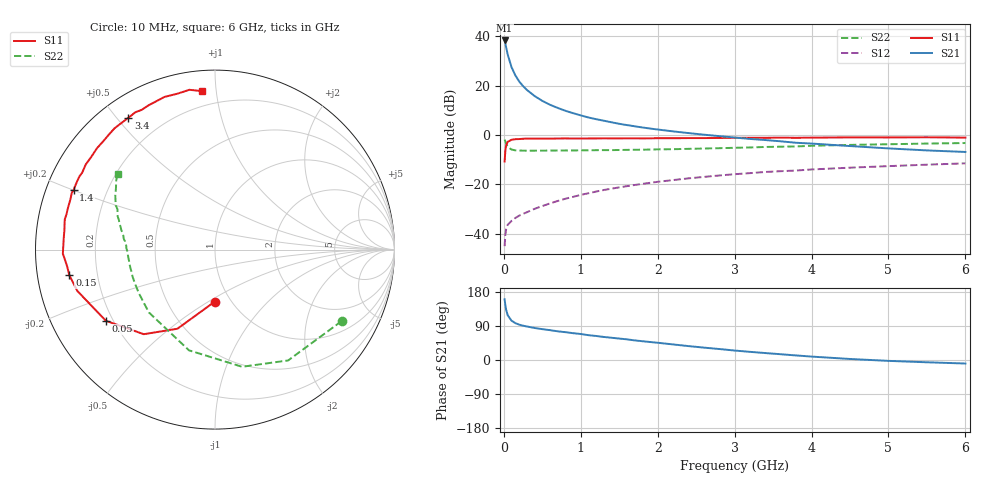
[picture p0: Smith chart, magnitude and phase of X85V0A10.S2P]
! SIEMENS Small Signal Semiconductors
! BFP136W
! Si NPN RF Bipolar Junction Transistor in SOT343
! VCE = 5 V  IC = 100 mA
! Common Emitter S-Parameters:  September  1994
# GHz  S  MA  R  50
!  f  S11  S21  S12  S22
! GHz  MAG  ANG  MAG  ANG  MAG  ANG  MAG  ANG
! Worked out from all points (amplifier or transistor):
!   40 points, 10 MHz to 6 GHz, reference 50 ohm
!   highest |S21| = 38.3 dB at 10 MHz (marker M1)
!   |S21| within 3 dB of that: start of sweep to 31.55 MHz
!   unconditionally stable (mu >= 1): 560.7 MHz to 2.921 GHz
!   at 200 MHz: K = 0.67, MSG = 27.2 dB, |S12| = -32.7 dB
!   at 1.5 GHz: K = 1.10, MAG = 11.0 dB, |S12| = -21.2 dB
!   at 6 GHz: K = 0.96, MSG = 2.3 dB, |S12| = -11.5 dB
!   S11 on the Smith chart (normalised r, x): 10 MHz: 0.84, -0.53; 50 MHz: 0.17, -0.29; 150 MHz: 0.10, -0.09; 1.4 GHz: 0.08, +0.20; 3.4 GHz: 0.08, +0.54; 6 GHz: 0.11, +0.91
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0.01  0.2904 -90.4  82.47 160.4  0.0056 69.8  0.81 -29.5
0.02  0.4881 -115.4  70.93 144.0  0.0097 57.5  0.7398 -56.6
0.03  0.6162 -130.1  59.92 132.4  0.0124 48.9  0.67 -77.0
0.05  0.726 -146.9  42.83 118.2  0.0152 40.2  0.5796 -104.5
0.1  0.801 -163.3  23.7 103.7  0.0182 36.7  0.5082 -136.5
0.15  0.824 -170.0  16.14 97.3  0.0209 38.9  0.489 -150.0
0.2  0.8292 -173.6  12.15 93.3  0.0233 40.6  0.4843 -157.3
0.25  0.84 -176.7  9.795 90.5  0.0253 43.5  0.4833 -161.9
0.3  0.848 -178.4  8.195 88.4  0.0273 45.7  0.4816 -165.1
0.4  0.8452 177.8  6.174 84.5  0.032 49.9  0.4826 -169.4
0.5  0.8453 174.8  4.924 81.4  0.0364 52.6  0.4831 -172.3
0.6  0.8457 172.8  4.107 78.8  0.0412 54.8  0.4841 -174.2
0.7  0.8503 170.3  3.542 75.7  0.0461 56.7  0.4857 -175.6
0.9  0.8503 166.6  2.772 70.8  0.0559 58.2  0.4877 -178.3
1.1  0.8519 162.2  2.268 65.5  0.0662 59.1  0.4909 -179.9
1.4  0.8544 157.1  1.811 58.7  0.0819 59.1  0.4947 177.6
2.2  0.8614 143.2  1.185 41.1  0.1223 54.4  0.5162 171.5
3.2  0.8771 126.2  0.834 21.5  0.1691 45.4  0.5601 162.9
3.4  0.879 123.3  0.791 18.3  0.1785 43.3  0.5732 161.1
4.5  0.896 108.3  0.598 2.7  0.2182 33.4  0.6313 151.6
5.5  0.9017 99.1  0.488 -6.0  0.2509 25.7  0.672 145.0
6  0.8861 94.8  0.454 -9.3  0.267 21.4  0.6881 142.0
